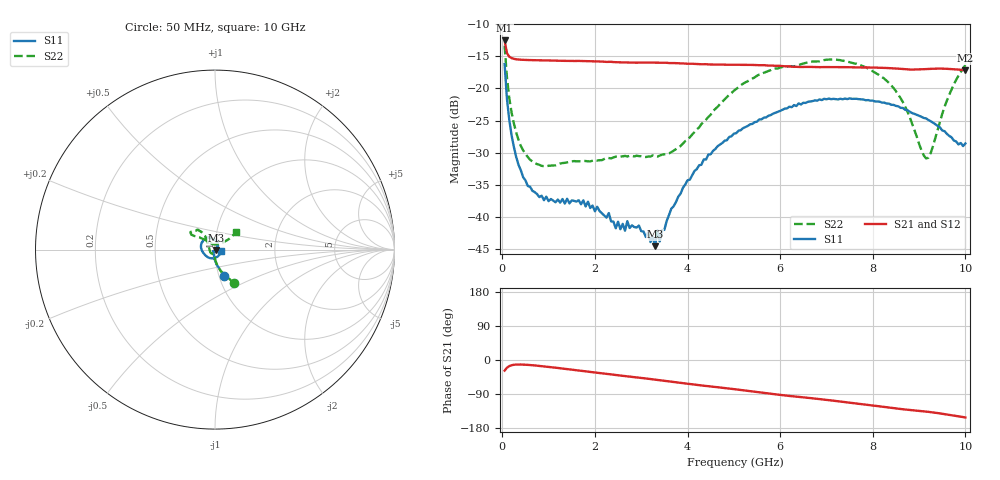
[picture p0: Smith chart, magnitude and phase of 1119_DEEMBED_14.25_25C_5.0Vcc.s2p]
!Hittite Microwave Corp.
!Digital Attenuator/PhaseShifter Rev 1.4.0
!Filename: C:\DATA\DATA\1119_DEEMBED_14.25_25C_5.0Vcc.s2p
!VNA ID: Agilent Technologies,N5224A,MY51441122,A.10.45.03
!Device type:
!2 Port Calibration.
!Temp(C): 25
!Lot Number:
!Serial Number:
!Operator:
!Misc:
!Attenuator:  14.250
# GHZ S DB R 50.0
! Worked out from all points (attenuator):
!   200 points, 50 MHz to 10 GHz, reference 50 ohm
!   highest |S21| = -12.52 dB at 50 MHz (marker M1); lowest = -17.2 dB at 10 GHz (marker M2)
!   lowest |S11| = -44.6 dB at 3.3 GHz (marker M3), VSWR 1.01, Z = 50.5 - j0.245 ohm
!   |S11| at or under -10 dB: start of sweep to end of sweep
!   |S22| runs from -32.1 to -13.3 dB; largest |S21 - S12| = 0.00056
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0.05  -16.20 -70.9  -12.52 -28.0  -12.52 -28.1  -13.33 -60.5
0.1  -21.59 -84.0  -14.47 -20.5  -14.47 -20.5  -18.23 -75.3
0.2  -27.28 -95.7  -15.27 -13.8  -15.27 -13.8  -23.74 -86.7
0.35  -31.90 -106.1  -15.49 -11.9  -15.49 -11.9  -28.02 -93.7
0.55  -35.20 -118.9  -15.57 -12.9  -15.57 -12.9  -30.68 -99.9
0.9  -37.41 -130.3  -15.63 -16.9  -15.63 -16.9  -32.11 -106.2
1.75  -37.43 -134.6  -15.73 -29.1  -15.73 -29.1  -31.28 -115.9
2.3  -39.42 -126.7  -15.85 -37.4  -15.85 -37.4  -30.85 -131.2
2.45  -41.79 -115.7  -15.91 -39.6  -15.91 -39.7  -30.63 -134.5
2.95  -41.37 -78.9  -15.96 -46.5  -15.97 -46.6  -30.55 -153.1
3.3  -44.58 -24.2  -15.98 -52.0  -15.99 -52.0  -30.55 -171.2
3.35  -42.11 -12.0  -15.99 -52.7  -16.00 -52.7  -30.62 -173.6
3.4  -43.85 -8.5  -15.99 -53.4  -16.00 -53.4  -30.47 -175.8
3.65  -38.73 25.3  -16.05 -57.3  -16.06 -57.3  -29.93 170.3
4  -34.31 43.1  -16.15 -62.7  -16.16 -62.7  -28.01 150.3
5.05  -26.98 77.2  -16.31 -77.6  -16.33 -77.6  -20.08 125.9
6.7  -21.97 127.5  -16.65 -101.2  -16.66 -101.2  -15.81 139.8
7.65  -21.61 157.7  -16.71 -114.8  -16.72 -114.8  -16.16 147.8
8.35  -22.37 178.2  -16.83 -125.5  -16.83 -125.5  -19.14 142.1
9.2  -24.92 -127.5  -16.96 -136.8  -16.97 -136.8  -30.81 81.3
9.6  -27.07 -83.8  -16.94 -143.9  -16.95 -143.9  -21.90 38.4
10  -28.57 -16.2  -17.18 -151.5  -17.19 -151.5  -16.36 39.6
